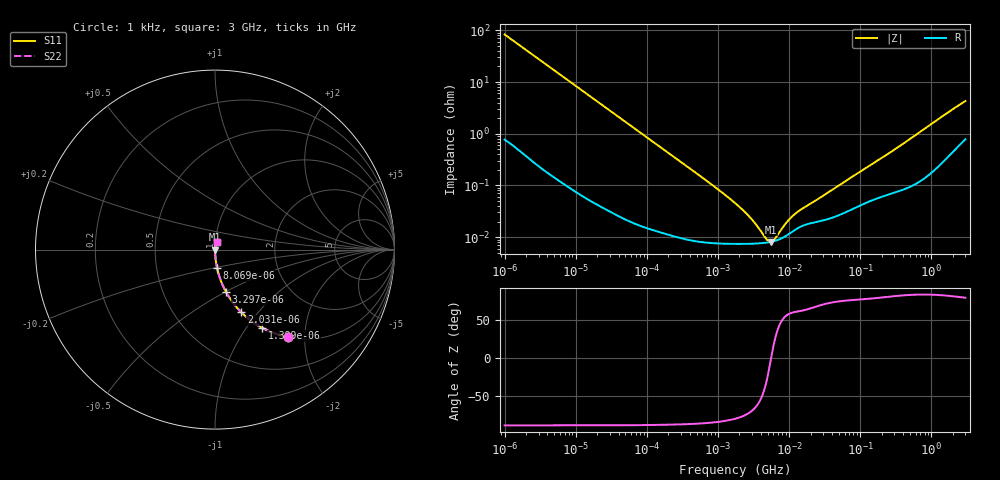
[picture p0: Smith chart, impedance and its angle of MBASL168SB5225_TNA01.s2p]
! MBASL168SB5225_TNA01  S-PARAMETER MODEL  ( Standard Model )
! Model Generated by TAIYO YUDEN Corporation (http://www.ty-top.com)
! Version 1.0
! TAIYO YUDEN Control No. 220601
! Copyright(c) 2012 TAIYO YUDEN CO.,LTD. All Rights Reserved.
! Product Description (link to TY-COMPAS)
! https://ds.yuden.co.jp/TYCOMPAS/or/detail?pn=MBASL168SB5225KTNA01&u=M
! Products Name : Multilayer Ceramic Capacitors
! Characteristics :
!  Capacitance : 2.2 [uF] , Rated Voltage : 10 [V] , TCC : X5R
!  Case Size : 1.6 x 0.8 / 0.063 x 0.031 [mm/inch] , Thickness : 0.8 / 0.031 [mm/inch]
!  (Conditions: Temperature = 25 [degC] , DC Bias Voltage = 0 [V])
! External Node Assignments :
!  1  o---| |---o  2
! GND o---------o GND
! Frequency Range : 1kHz  -  3GHz  [ 401 STEP ]
# MHZ S RI R 50
! Freq[MHz].  S11 Real  S11 Imag  S21 Real  S21 Imag  S12 Real  S12 Imag  S22 Real  S22 Imag
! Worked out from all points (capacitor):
!   401 points, 1 kHz to 3 GHz, reference 50 ohm
!   read as one part in series: C = 1.91 uF near 1.077 kHz
!   lowest |Z| = 8.09 mohm at 5.502 MHz (marker M1)
!   series resonance near 5.582 MHz, so ESL is about 430 pH
!   S11 on the Smith chart (normalised r, x): 1 kHz: 1.02, -1.66; 1.399 kHz: 1.01, -1.19; 2.031 kHz: 1.01, -0.82; 3.297 kHz: 1.00, -0.51; 8.069 kHz: 1.00, -0.21; 3 GHz: 1.02, +0.08
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0.001  0.4093 -0.4871  0.5907 0.4871  0.5907 0.4871  0.4093 -0.4871
0.001399  0.2638 -0.4361  0.7362 0.4361  0.7362 0.4361  0.2638 -0.4361
0.002031  0.1468 -0.3496  0.8532 0.3496  0.8532 0.3496  0.1468 -0.3496
0.003297  0.0623 -0.2375  0.9377 0.2375  0.9377 0.2375  0.0623 -0.2375
0.008069  0.0116 -0.1029  0.9884 0.1029  0.9884 0.1029  0.0116 -0.1029
0.01216  0.0054 -0.0689  0.9946 0.0689  0.9946 0.0689  0.0054 -0.0689
0.033275  0.000937 -0.0254  0.9991 0.0254  0.9991 0.0254  0.000937 -0.0254
0.147855  0.000159 -0.00577  0.9998 0.00577  0.9998 0.00577  0.000159 -0.00577
0.762639  7.85e-05 -0.00111  0.9999 0.00111  0.9999 0.00111  7.85e-05 -0.00111
1.732051  7.42e-05 -0.000451  0.9999 0.000451  0.9999 0.000451  7.42e-05 -0.000451
2.812335  7.44e-05 -0.00023  0.9999 0.00023  0.9999 0.00023  7.44e-05 -0.00023
4.399271  7.71e-05 -7.51e-05  0.9999 7.51e-05  0.9999 7.51e-05  7.71e-05 -7.51e-05
4.739869  7.8e-05 -5.14e-05  0.9999 5.14e-05  0.9999 5.14e-05  7.8e-05 -5.14e-05
5.502215  8.07e-05 -4.46e-06  0.9999 4.46e-06  0.9999 4.46e-06  8.07e-05 -4.46e-06
6.629817  8.64e-05 5.43e-05  0.9999 -5.43e-05  0.9999 -5.43e-05  8.64e-05 5.43e-05
8.933959  0.000105 0.000151  0.9999 -0.000151  0.9999 -0.000151  0.000105 0.000151
11.1738  0.000129 0.000222  0.9999 -0.000222  0.9999 -0.000222  0.000129 0.000222
13.97519  0.000155 0.000289  0.9998 -0.000289  0.9998 -0.000289  0.000155 0.000289
21.06097  0.000188 0.000425  0.9998 -0.000425  0.9998 -0.000425  0.000188 0.000425
256.0921  0.000689 0.00417  0.9993 -0.00417  0.9993 -0.00417  0.000689 0.00417
1652.1  0.004 0.0246  0.996 -0.0246  0.996 -0.0246  0.004 0.0246
3000  0.00951 0.0415  0.9905 -0.0415  0.9905 -0.0415  0.00951 0.0415
